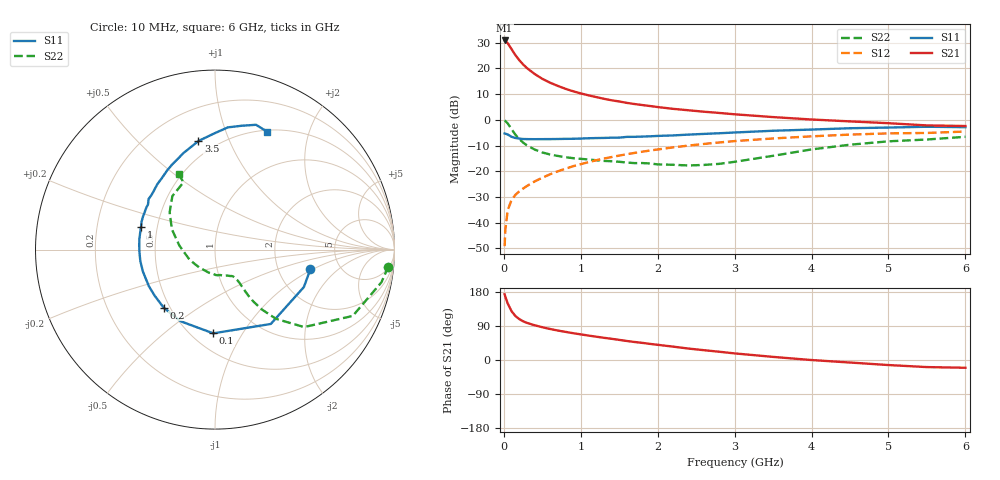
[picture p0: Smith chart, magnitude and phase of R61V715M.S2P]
! SIEMENS Small Signal Semiconductors
! BFR193
! Si NPN RF Bipolar Junction Transistor in SOT23
! VCE = 1.75 V  IC = 15 mA
! Common Emitter S-Parameters:  May  1996
# GHz  S  MA  R  50
!  f  S11  S21  S12  S22
! GHz  MAG  ANG  MAG  ANG  MAG  ANG  MAG  ANG
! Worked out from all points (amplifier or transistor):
!   36 points, 10 MHz to 6 GHz, reference 50 ohm
!   highest |S21| = 30.8 dB at 10 MHz (marker M1)
!   |S21| within 3 dB of that: start of sweep to 91.88 MHz
!   unconditionally stable (mu >= 1): 592.8 MHz to 1.964 GHz
!   at 250 MHz: K = 0.77, MSG = 24.1 dB, |S12| = -26.7 dB
!   at 1.4 GHz: K = 1.03, MAG = 9.9 dB, |S12| = -14.5 dB
!   at 6 GHz: K = 0.95, MSG = 1.1 dB, |S12| = -4.6 dB
!   S11 on the Smith chart (normalised r, x): 10 MHz: 3.04, -0.95; 100 MHz: 0.63, -0.75; 200 MHz: 0.46, -0.37; 1 GHz: 0.40, +0.13; 3.5 GHz: 0.40, +0.78; 6 GHz: 0.52, +1.40
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0.01  0.5423 -11.7  34.77 173.3  0.0035 85.5  0.97 -5.6
0.02  0.5375 -22.8  34.17 166.6  0.0074 80.3  0.9451 -11.1
0.05  0.518 -53.1  30.78 149.3  0.0175 70.4  0.8519 -25.7
0.1  0.4667 -91.2  23.57 128.9  0.0276 62.3  0.658 -41.0
0.15  0.4428 -115.7  18.07 116.1  0.0348 58.8  0.5145 -48.6
0.2  0.4317 -131.6  14.45 108.1  0.0406 58.7  0.4244 -51.9
0.25  0.423 -142.7  11.91 102.2  0.046 59.7  0.3612 -53.5
0.3  0.4211 -151.2  10.11 98.0  0.0517 61.5  0.318 -54.1
0.4  0.4199 -163.1  7.757 91.7  0.0633 63.6  0.2644 -54.0
0.5  0.4209 -171.2  6.253 86.5  0.0748 64.8  0.2316 -53.6
0.6  0.4212 -178.1  5.264 81.9  0.0871 65.7  0.2117 -53.8
0.7  0.4231 176.4  4.56 77.8  0.0995 66.1  0.1985 -54.3
0.8  0.4255 171.9  4.006 74.3  0.1121 65.8  0.1871 -55.3
1  0.4316 162.7  3.251 67.6  0.1374 65.1  0.1742 -57.7
1.1  0.4378 159.0  2.985 64.5  0.1503 64.4  0.1693 -60.4
1.3  0.4437 152.2  2.56 58.6  0.1766 62.6  0.1589 -65.2
1.6  0.4653 142.7  2.129 50.1  0.2145 59.5  0.1474 -76.0
2.2  0.4964 126.6  1.631 35.3  0.2905 51.9  0.1334 -104.2
3.5  0.6119 98.7  1.128 8.2  0.4335 32.4  0.1995 173.7
4.5  0.6848 84.0  0.93 -6.7  0.5154 17.8  0.3278 140.4
5.5  0.732 71.8  0.777 -18.7  0.5545 3.2  0.4136 115.1
6  0.7184 66.2  0.757 -20.5  0.5904 -1.1  0.4668 115.7
